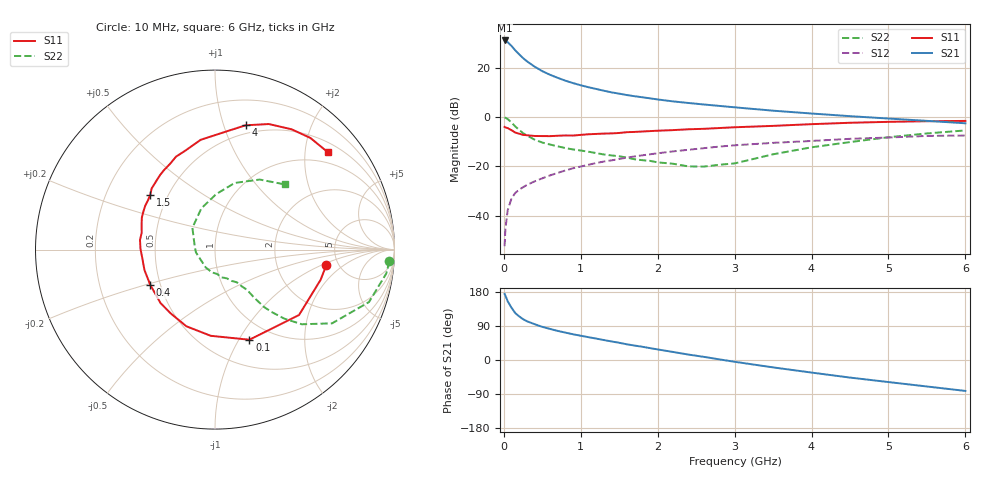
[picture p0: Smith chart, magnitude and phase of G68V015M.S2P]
! SIEMENS Small Signal Semiconductors
! BFG193
! Si NPN RF Bipolar Junction Transistor in SOT223
! VCE = 8 V  IC = 15 mA
! Common Emitter S-Parameters:  August  1996
# GHz  S  MA  R  50
!  f  S11  S21  S12  S22
! GHz  MAG  ANG  MAG  ANG  MAG  ANG  MAG  ANG
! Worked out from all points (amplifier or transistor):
!   36 points, 10 MHz to 6 GHz, reference 50 ohm
!   highest |S21| = 31.0 dB at 10 MHz (marker M1)
!   |S21| within 3 dB of that: start of sweep to 121.1 MHz
!   unconditionally stable (mu >= 1): 805.4 MHz to 2.553 GHz
!   at 250 MHz: K = 0.65, MSG = 26.2 dB, |S12| = -28.5 dB
!   at 1.4 GHz: K = 1.06, MAG = 12.3 dB, |S12| = -17.6 dB
!   at 6 GHz: K = 0.87, MSG = 2.5 dB, |S12| = -7.5 dB
!   S11 on the Smith chart (normalised r, x): 10 MHz: 4.03, -1.11; 100 MHz: 0.79, -1.11; 400 MHz: 0.44, -0.21; 1.5 GHz: 0.40, +0.31; 4 GHz: 0.42, +1.19; 6 GHz: 0.72, +2.51
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0.01  0.6266 -7.7  35.47 174.3  0.0024 88.3  0.9734 -3.9
0.02  0.6122 -15.9  34.97 170.1  0.0053 80.8  0.9638 -7.9
0.05  0.5933 -37.9  32.77 155.1  0.0128 73.0  0.9065 -18.8
0.1  0.5375 -69.1  27.45 137.7  0.0224 65.3  0.7709 -32.2
0.15  0.4809 -92.8  22.22 123.5  0.0289 58.1  0.6379 -40.7
0.2  0.4561 -110.5  18.51 115.0  0.0337 56.9  0.5447 -44.9
0.25  0.4328 -124.7  15.58 107.8  0.0376 55.6  0.4689 -47.8
0.3  0.4254 -135.5  13.43 102.3  0.0417 55.2  0.4199 -49.5
0.4  0.4107 -151.5  10.44 94.5  0.0494 56.2  0.3462 -50.8
0.5  0.4092 -163.9  8.463 87.4  0.057 56.8  0.3022 -51.3
0.6  0.4078 -173.1  7.151 82.0  0.0653 57.2  0.2757 -52.2
0.7  0.4152 179.4  6.196 76.8  0.0734 56.9  0.2534 -53.9
0.9  0.4191 167.0  4.848 67.9  0.0912 55.6  0.2191 -56.3
1.1  0.445 156.3  4 60.2  0.1072 53.7  0.1972 -62.3
1.5  0.4728 139.7  2.965 45.4  0.1404 47.6  0.1593 -76.7
2.2  0.5404 117.4  2.064 21.2  0.2001 34.6  0.1125 -117.1
2.8  0.5952 101.7  1.672 1.7  0.2503 22.1  0.1072 -171.5
3.5  0.6583 85.1  1.338 -19.5  0.2982 5.8  0.1748 136.1
4  0.7131 76.2  1.172 -33.2  0.3257 -3.7  0.2422 108.3
4.5  0.7611 66.8  1.036 -46.4  0.3598 -13.9  0.3091 88.8
5.5  0.8182 49.5  0.832 -69.9  0.4119 -37.6  0.4628 57.5
6  0.8304 40.8  0.743 -81.6  0.4202 -51.4  0.5323 43.0
